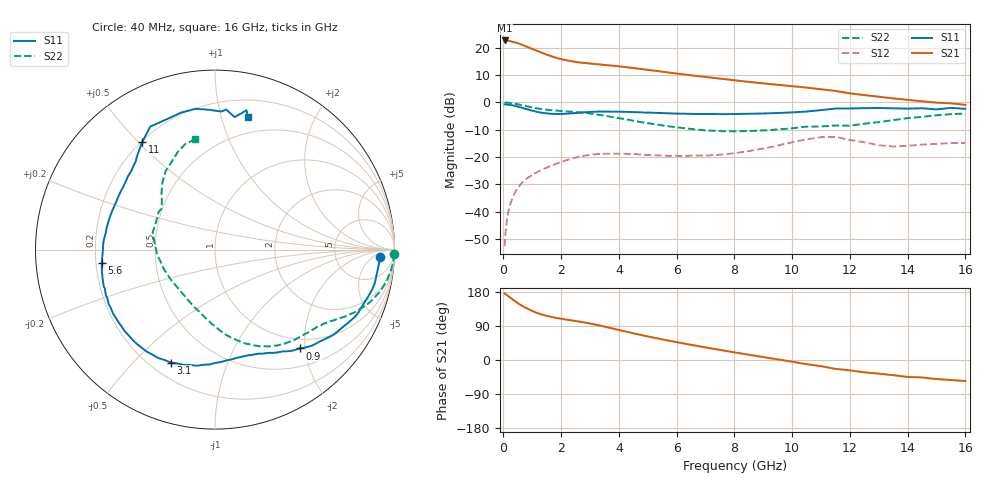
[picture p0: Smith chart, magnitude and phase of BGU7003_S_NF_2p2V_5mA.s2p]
!	Filename:	P:\Prog\Test\Noise\ATS_data\Testdata_Net\BGU7002	BGU7003	RN20082092\BGU7003_B1_high	freq_bias	loop_2.2V4.55mA_D.s2p
!	Date/Time:	Tue	16-Sep-08	9:21:28
!	BGU7003_B1_high	freq_bias	loop
!	bias	mode	1:00	Vout=	2.2	"V,"	Iout=	4.6	"mA,"	Vin=	2.467	"V,"	Iin=	0.4845	mA
!	Date/time	Sun	Aug	10	19:09:55	2008
!	Device	data	file	deembeded	for	feedlines	and	parallel
!	Original	file:	\BGU7002	BGU7003	RN20082092\BGU7003_B1_high	freq_bias	loop_2.2V4.55mA_R.s2p
!	Feed-files:	PR029V01_high	"frequency_140808_Feed1.s2p,"	PR029V01_high	frequency_140808_Feed2.s2p
!	Parallel-file:	PR029V01_high	frequency_140808_Par.s2p
#	MHz	S	MA	R	50
!	Freq-MHz	S11-mag	S11-arg	S21-mag	S21-arg	S12-mag	S12-arg	S22-mag	S22-arg
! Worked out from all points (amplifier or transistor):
!   148 points, 40 MHz to 16 GHz, reference 50 ohm
!   highest |S21| = 22.7 dB at 50 MHz (marker M1)
!   |S21| within 3 dB of that: start of sweep to 974.9 MHz
!   unconditionally stable (mu >= 1): nowhere
!   at 280 MHz: K = 0.14, MSG = 29.1 dB, |S12| = -35.9 dB
!   at 1.95 GHz: K = 0.50, MSG = 19.0 dB, |S12| = -22.0 dB
!   at 16 GHz: K = 0.86, MSG = 7.0 dB, |S12| = -14.9 dB
!   lowest NFmin = 0.45 dB at 400 MHz
!   S11 on the Smith chart (normalised r, x): 40 MHz: 19, -10; 900 MHz: 0.81, -1.90; 3.1 GHz: 0.28, -0.65; 5.6 GHz: 0.22, -0.06; 11 GHz: 0.20, +0.51; 16 GHz: 0.34, +1.22
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40  0.9215 -2.6  13.69 176.0  0.00232 86.2  0.9979 -1.4
50  0.9199 -3.2  13.69 175.2  0.00286 85.5  0.9974 -1.8
130  0.912 -8.5  13.55 170.8  0.00759 84.5  0.9924 -4.8
230  0.9012 -14.9  13.31 164.9  0.01327 81.3  0.9804 -8.5
470  0.8443 -29.1  12.32 151.5  0.02579 73.5  0.9317 -16.2
650  0.7962 -38.3  11.36 142.6  0.03393 68.8  0.888 -21.0
900  0.7269 -49.2  10.05 132.7  0.04358 63.8  0.8275 -26.0
1100  0.6819 -56.2  9.086 126.0  0.05056 60.9  0.7872 -29.1
1300  0.6497 -62.2  8.235 120.7  0.05732 58.5  0.7565 -31.8
1650  0.6207 -71.2  7.061 113.7  0.06934 54.6  0.7197 -36.3
2100  0.6193 -82.3  6.049 107.5  0.08484 48.9  0.69 -42.5
2700  0.6549 -98.9  5.369 100.5  0.1035 39.0  0.6538 -53.0
3100  0.6753 -111.3  5.121 94.8  0.1114 31.7  0.6181 -60.9
4300  0.6706 -146.1  4.402 74.0  0.1144 15.8  0.4831 -81.9
5400  0.6414 -169.4  3.72 55.9  0.1071 10.8  0.3863 -97.6
5600  0.6354 -173.2  3.602 52.9  0.1054 10.5  0.3713 -100.6
6800  0.6158 168.3  3.015 35.9  0.1062 11.9  0.3144 -120.2
8200  0.6148 150.4  2.488 17.6  0.1215 17.7  0.2976 -146.2
9600  0.6426 136.0  2.082 0.4  0.1672 16.0  0.3246 -175.8
11000  0.7231 124.2  1.744 -16.3  0.2307 -5.5  0.3631 154.3
13500  0.7812 93.1  1.184 -40.0  0.1557 -29.5  0.4741 128.3
16000  0.7635 76.2  0.9016 -55.5  0.1801 -38.9  0.6254 100.1
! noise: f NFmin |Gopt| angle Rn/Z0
400  0.45  0.42  8.59  0.16
1000  0.57  0.4  24.27  0.17
1500  0.66  0.39  37.33  0.17
1700  0.7  0.38  42.56  0.17
2200  0.79  0.37  55.62  0.16
3000  0.94  0.36  76.52  0.15
4400  1.21  0.35  113.1  0.12
5800  1.47  0.36  149.7  0.09
8000  1.88  0.41  -162.5  0.08
1.2e+04  2.63  0.59  -123.5  0.37
